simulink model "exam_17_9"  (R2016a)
settings: Solver=ode23tb  StartTime=0.0  StopTime=0.02  RelTol=1e-3
libraries: powerlib x13

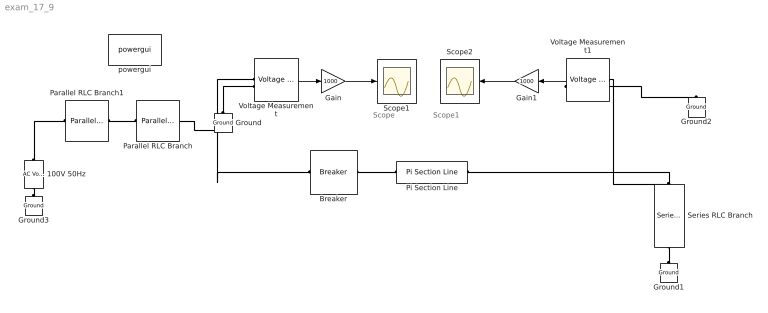
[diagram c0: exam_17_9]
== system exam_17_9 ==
  note: Scope1
  note: Scope
  100V 50Hz : powerlib/Electrical Sources/AC Voltage Source  Amplitude=100  Phase=0  Frequency=50  SampleTime=0  Measurements=None  BusType=swing  Pref=10e3  Qref=0  Qmin=-inf  Qmax=+inf
  Breaker : powerlib/Elements/Breaker  InitialState=0  SwitchingTimes="[1/200  5/200]"  External=off  BreakerResistance=0.001  SnubberResistance=inf  SnubberCapacitance=0  Measurements=None  MoreParameters=on  NoBreakLoop=off
  Gain : Gain  Gain=1000
  Gain1 : Gain  Gain=1000
  Ground{,1..3} (4 alike) : powerlib/Elements/Ground  LConnTagsString=a
  Parallel RLC Branch : powerlib/Elements/Parallel RLC Branch  LConnTagsString=a  RConnTagsString=__new0  BranchType=RLC  Resistance=180.1  Inductance=26.525e-3  SetiL0=off  InitialCurrent=0  Capacitance=117.84e-6  Setx0=off  InitialVoltage=0  Measurements=None
  Parallel RLC Branch1 : powerlib/Elements/Parallel RLC Branch  LConnTagsString=a  RConnTagsString=__new0  BranchType=R  Resistance=1  Inductance=1e-3  SetiL0=off  InitialCurrent=0  Capacitance=1e-6  Setx0=off  InitialVoltage=0  Measurements=None
  Pi Section Line : powerlib/Elements/Pi Section Line  LConnTagsString=__new0  RConnTagsString=__new0  Frequency=50  Resistance=0.1  Inductance=0.0016  Capacitance=0.0102e-6  Length=300  PiSections=10  Measurements=None
  Scope1 : Scope
  Scope2 : Scope
  Series RLC Branch : powerlib/Elements/Series RLC Branch  LConnTagsString=__new0  RConnTagsString=__new0  BranchType=RL  Resistance=1  Inductance=1  SetiL0=off  InitialCurrent=0  Capacitance=3.06e-6  Setx0=off  InitialVoltage=0  Measurements=None
  Voltage Measurement : powerlib/Measurements/Voltage Measurement  PhasorSimulation=off  OutputType=Complex  PSBequivalent=0
  Voltage Measurement1 : powerlib/Measurements/Voltage Measurement  PhasorSimulation=off  OutputType=Complex  PSBequivalent=0
  powergui : powerlib/powergui  Priority=1  SimulationMode=Continuous  SolverType=Tustin  SampleTime=25e-6  frequency=60  SPID=off  DisableSnubberDevices=off  DisableRonSwitches=off  DisableVfSwitches=off  SwTol=0  DisplayEquations=off  Interpol=off  ExternalGateDelay=off  methode=off  Ts=10  FunctionMessages=off  echomessages=off  HookPort=off  EnableUseOfTLC=off  x0status=blocks  frequencyindice=50  Pbase=100e6  ErrMax=1e-4  Iterations=50  UnitsV=kV  UnitsW=MW  buscounter=0  RestoreLinks=warning  ResistiveCurrentMeasurement=off  Frange=[0:2:500]  Ylog=on  Xlog=off  ShowGrid=on  save=off  variable=ZData  structure=0  ZoomFFT=off  StartTime=0.0  cycles=1  DisplayStyle=1  fundamental=60  FreqAxis=off  MaxFrequency=1000  frequencyindicesteady=1  RmsSteady=1  display=off
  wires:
  Voltage Measurement/1 -> Gain/1
  Gain/1 -> Scope1/1
  Gain1/1 -> Scope2/1
  Voltage Measurement1/1 -> Gain1/1
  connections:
  Voltage Measurement/LConn1 -- Parallel RLC Branch/RConn1 -- Breaker/LConn1
  Series RLC Branch/LConn1 -- Voltage Measurement1/LConn1 -- Pi Section Line/RConn1
  Ground/LConn1 -- Voltage Measurement/LConn2
  Series RLC Branch/RConn1 -- Ground1/LConn1
  Breaker/RConn1 -- Pi Section Line/LConn1
  Ground3/LConn1 -- 100V 50Hz/LConn1
  Voltage Measurement1/LConn2 -- Ground2/LConn1
  Parallel RLC Branch1/LConn1 -- Parallel RLC Branch/LConn1
  100V 50Hz/RConn1 -- Parallel RLC Branch1/RConn1
